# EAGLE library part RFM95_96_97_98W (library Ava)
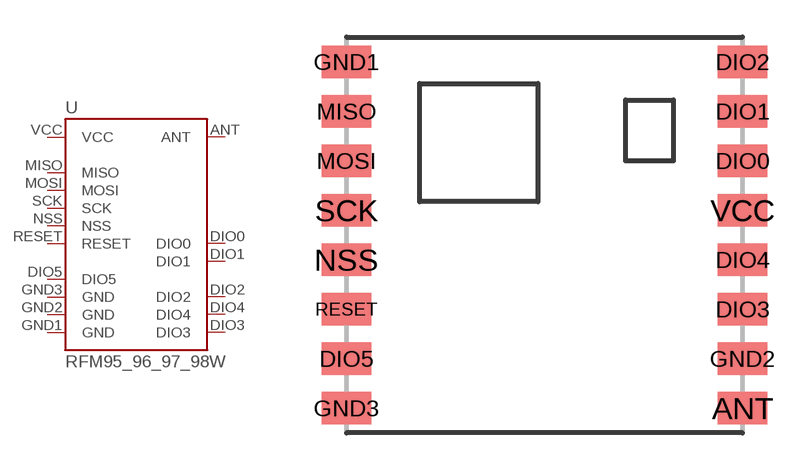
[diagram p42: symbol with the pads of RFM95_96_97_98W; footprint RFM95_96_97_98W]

Designator prefix -

## RFM95_96_97_98W  [RFM95_96_97_98W]
ANT  ANT
DIO0  DIO0  in
DIO1  DIO1  in
DIO2  DIO2
DIO3  DIO3
DIO4  DIO4
DIO5  DIO5  in
GND1  GND  pwr
GND2  GND  pwr
GND3  GND  pwr
MISO  MISO  out
MOSI  MOSI  in
NSS  NSS  in
RESET  RESET  out
SCK  SCK  in
VCC  VCC

## Footprint RFM95_96_97_98W (pad centres in mm)
smd 2 x 1.3: ANT 8,-7; DIO0 8,3; DIO1 8,5; DIO2 8,7; DIO3 8,-3; DIO4 8,-1; DIO5 -8,-5; GND1 -8,7; GND2 8,-5; GND3 -8,-7; MISO -8,5; MOSI -8,3; NSS -8,-1; RESET -8,-3; SCK -8,1; VCC 8,1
